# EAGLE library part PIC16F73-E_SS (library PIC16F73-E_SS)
Microchip PIC16F73-E/SS, 8bit PIC Microcontroller, 20MHz, 4096 B Flash, 28-Pin SSOP Source: Datasheet
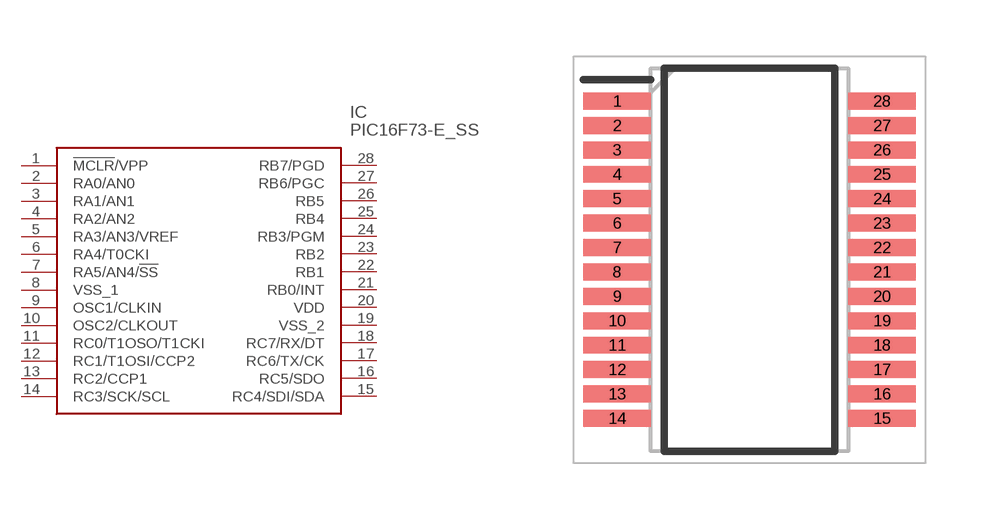
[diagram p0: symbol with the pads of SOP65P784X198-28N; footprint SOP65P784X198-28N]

Designator prefix IC

## PIC16F73-E_SS (Description: Microchip PIC16F73-E/SS, 8bit PIC Microcontroller, 20MHz, 4096 B Flash, 28-Pin SSOP; Height: 1.98mm; Manufacturer_Name: Microchip; Manufacturer_Part_Number: PIC16F73-E/SS; Mouser_Part_Number: 579-PIC16F73-E/SS; Mouser_Price-Stock: https://www.mouser.co.uk/ProductDetail/Microchip-Technology-Atmel/PIC16F73-E-SS?qs=iRhCjdSJZe7qYox7WGvMBA%3D%3D)  [SOP65P784X198-28N]
1  !MCLR!/VPP
2  RA0/AN0
3  RA1/AN1
4  RA2/AN2
5  RA3/AN3/VREF
6  RA4/T0CKI
7  RA5/AN4/!SS
8  VSS_1
9  OSC1/CLKIN
10  OSC2/CLKOUT
11  RC0/T1OSO/T1CKI
12  RC1/T1OSI/CCP2
13  RC2/CCP1
14  RC3/SCK/SCL
15  RC4/SDI/SDA
16  RC5/SDO
17  RC6/TX/CK
18  RC7/RX/DT
19  VSS_2
20  VDD
21  RB0/INT
22  RB1
23  RB2
24  RB3/PGM
25  RB4
26  RB5
27  RB6/PGC
28  RB7/PGD

## Footprint SOP65P784X198-28N (pad centres in mm)
(SS)28-Lead(SSOP)-oldest
smd 1.8 x 0.45: 1 -3.525,4.225; 2 -3.525,3.575; 3 -3.525,2.925; 4 -3.525,2.275; 5 -3.525,1.625; 6 -3.525,0.975; 7 -3.525,0.325; 8 -3.525,-0.325; 9 -3.525,-0.975; 10 -3.525,-1.625; 11 -3.525,-2.275; 12 -3.525,-2.925; 13 -3.525,-3.575; 14 -3.525,-4.225; 15 3.525,-4.225; 16 3.525,-3.575; 17 3.525,-2.925; 18 3.525,-2.275; 19 3.525,-1.625; 20 3.525,-0.975; 21 3.525,-0.325; 22 3.525,0.325; 23 3.525,0.975; 24 3.525,1.625; 25 3.525,2.275; 26 3.525,2.925; 27 3.525,3.575; 28 3.525,4.225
